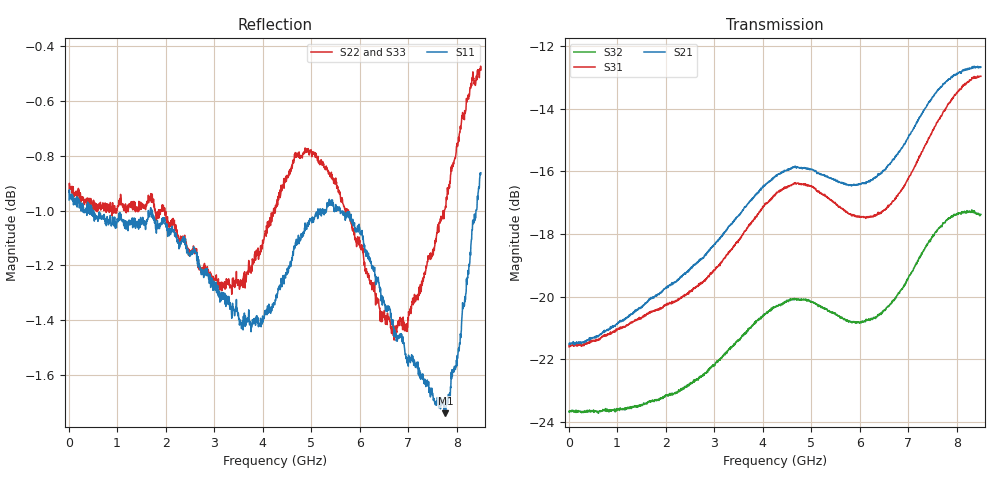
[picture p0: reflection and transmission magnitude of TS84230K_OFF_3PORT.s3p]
! Created with skrf (http://scikit-rf.org).
# Hz S RI R 50.0
!freq ReS11 ImS11 ReS12 ImS12 ReS13 ImS13
! ReS21 ImS21 ReS22 ImS22 ReS23 ImS23
! ReS31 ImS31 ReS32 ImS32 ReS33 ImS33
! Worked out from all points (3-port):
!   1601 points, 10 MHz to 8.5 GHz, reference 50 ohm
!   strongest paths, dB at 10 MHz, 2.132 GHz, 4.255 GHz, 6.378 GHz, 8.5 GHz:
!     S21: -21.5, -19.6, -16.2, -16.1, -12.7
!     S31: -21.6, -20.1, -16.8, -17.3, -13.0
!     S32: -23.7, -23.1, -20.3, -20.6, -17.4
!   lowest |S11| = -1.7 dB at 7.768 GHz (marker M1), VSWR 10.01, Z = 11.8 + j57.7 ohm
!   |S11| at or under -10 dB: nowhere
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1e7  -0.8953 0.00406  0.0841 -0.000161  0.0835 -0.000368
     0.0839 -0.000313  -0.8981 0.00503  0.0654 -0.000117
     0.0832 -0.000129  0.0655 -0.000261  -0.8988 0.00397
7.3165e8  -0.8677 0.197  0.088 0.00601  0.0866 0.00354
          0.0881 0.00598  -0.8534 0.2637  0.0658 -0.00396
          0.0868 0.0034  0.0658 -0.00414  -0.8581 0.2506
1.697388e9  -0.7811 0.4301  0.0992 0.0066  0.0946 0.00216
            0.0991 0.00684  -0.7232 0.5317  0.0677 -0.00939
            0.0947 0.0023  0.0676 -0.00931  -0.7213 0.5289
3.289262e9  -0.6058 0.6071  0.129 -0.00408  0.1173 -0.00359
            0.1287 -0.00445  -0.3673 0.782  0.0786 -0.0239
            0.1174 -0.00362  0.0785 -0.0238  -0.4352 0.7539
4.255e9  -0.3749 0.7714  0.1506 -0.0387  0.1419 -0.0332
         0.1508 -0.0384  -0.0363 0.8915  0.0829 -0.0492
         0.1414 -0.0331  0.0827 -0.0491  -0.1534 0.8759
5.364006e9  -0.0893 0.8887  0.1321 -0.0811  0.1211 -0.0766
            0.1322 -0.0805  0.2222 0.8781  0.0619 -0.0717
            0.1212 -0.0765  0.0622 -0.0716  0.1985 0.8827
6.382806e9  -0.0554 0.8648  0.1299 -0.0884  0.1136 -0.0751
            0.13 -0.0883  0.3507 0.7821  0.0565 -0.0747
            0.1138 -0.0751  0.0566 -0.0746  0.27 0.8413
7.088538e9  -0.0133 0.8365  0.1444 -0.1141  0.1316 -0.0881
            0.1444 -0.1138  0.529 0.6748  0.0596 -0.0924
            0.132 -0.0877  0.0596 -0.0921  0.3156 0.809
7.767738e9  0.1353 0.8071  0.1395 -0.1695  0.1454 -0.1361
            0.1401 -0.1689  0.7275 0.5175  0.0443 -0.1244
            0.1451 -0.1356  0.0443 -0.1241  0.4977 0.7206
8.5e9  0.4468 0.7876  0.0743 -0.2204  0.0918 -0.2053
       0.0754 -0.2197  0.8763 0.3552  -0.00997 -0.1343
       0.0925 -0.2047  -0.00921 -0.135  0.7769 0.5357
